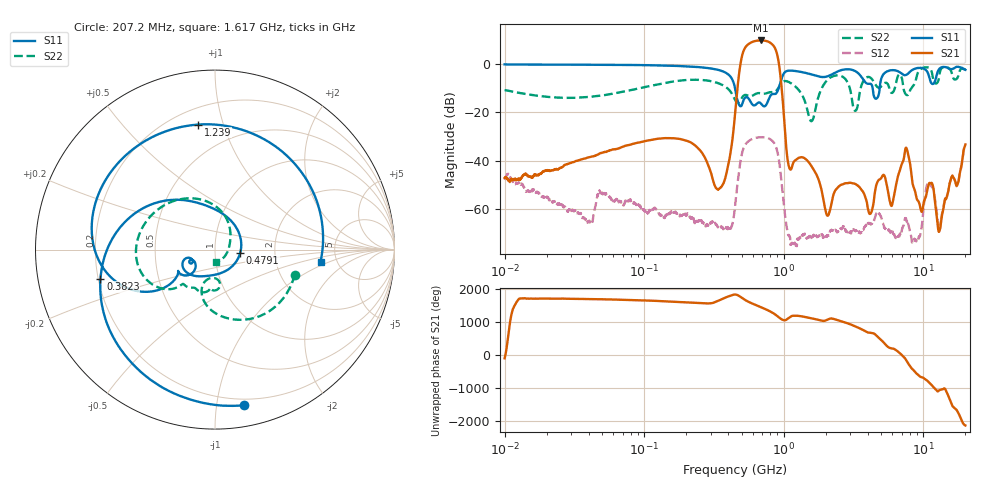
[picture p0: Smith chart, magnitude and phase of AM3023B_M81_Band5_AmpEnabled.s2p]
!Agilent Technologies,E8364B,MY43040894,A.07.50.67
!Agilent E8364B: A.07.50.67
!Date: Tuesday, October 27, 2020 10:43:54
!Correction: S11(Full 2 Port(1,2))
!S21(Full 2 Port(1,2))
!S12(Full 2 Port(1,2))
!S22(Full 2 Port(1,2))
!S2P File: Measurements: S11, S21, S12, S22:Log Frequency Sweep
# Hz S  dB  R 50
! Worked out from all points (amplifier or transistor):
!   3201 points, 10 MHz to 20 GHz, reference 50 ohm
!   highest |S21| = 9.6 dB at 684.2 MHz (marker M1)
!   |S21| within 3 dB of that: 528.3 MHz to 862.1 MHz (333.8 MHz wide, 48 % of centre)
!   unconditionally stable (mu >= 1): start of sweep to end of sweep
!   at 35.47 MHz: K = 5171.63, MAG = -28.6 dB, |S12| = -62.7 dB
!   at 447.2 MHz: K = 4408.85, MAG = -20.4 dB, |S12| = -59.1 dB
!   at 20 GHz: K = 203.75, MAG = -25.9 dB, |S12| = -33.8 dB
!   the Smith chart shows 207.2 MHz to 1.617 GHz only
!   S11 on the Smith chart (normalised r, x): 207.2 MHz: 0.15, -1.19; 382.3 MHz: 0.21, -0.12; 479.1 MHz: 1.33, -0.05; 1.239 GHz: 0.30, +0.83; 1.617 GHz: 3.73, -0.77
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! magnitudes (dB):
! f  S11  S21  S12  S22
! 10 MHz  -0.3  -47.1  -47.9  -10.9
! 35.55 MHz  -0.4  -39.5  -62.8  -13.9
! 126.1 MHz  -0.7  -30.9  -61.1  -8.4
! 207.2 MHz  -1.1  -32.0  -62.4  -6.6
! 382.3 MHz  -3.6  -46.8  -67.6  -9.5
! 447.2 MHz  -10.0  -21.0  -59.1  -14.9
! 479.1 MHz  -17.0  -3.7  -43.6  -15.7
! 684.2 MHz  -16.3  9.6  -30.3  -12.2
! 884.3 MHz  -12.1  5.1  -34.7  -11.1
! 1.08 GHz  -2.8  -41.5  -70.8  -7.4
! 1.239 GHz  -3.1  -39.4  -75.3  -9.9
! 1.59 GHz  -4.4  -42.5  -71.3  -23.6
! 1.617 GHz  -4.6  -43.2  -71.3  -22.9
! 2.06 GHz  -5.2  -62.6  -70.7  -6.6
! 3.25 GHz  -3.0  -49.6  -68.8  -19.4
! 4.586 GHz  -14.4  -50.3  -61.9  -9.0
! 5.639 GHz  -2.9  -54.2  -68.7  -9.2
! 7.588 GHz  -4.5  -35.0  -65.1  -12.9
! 9.22 GHz  -1.7  -56.8  -72.4  -3.2
! 10.97 GHz  -5.1  -49.4  -48.7  -1.6
! 13.04 GHz  -2.0  -69.0  -66.5  -4.4
! 20 GHz  -2.5  -33.3  -33.8  -2.3
